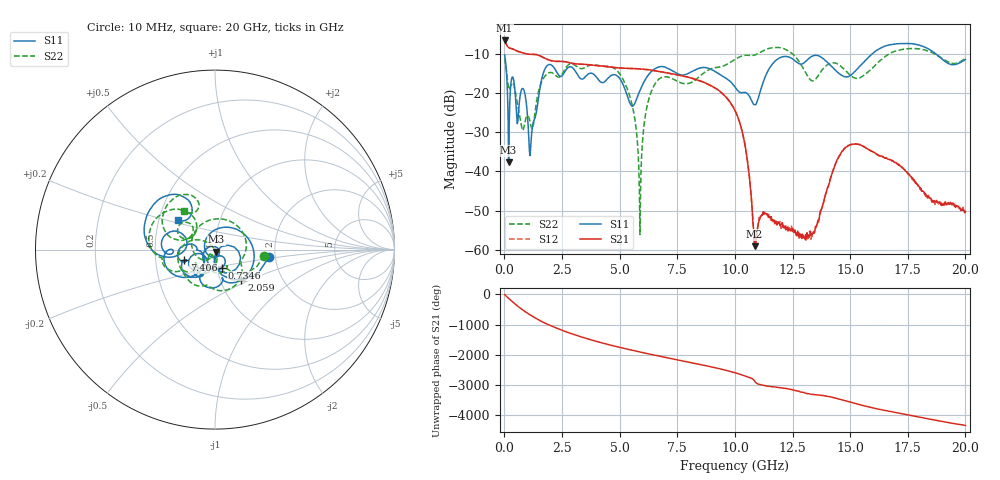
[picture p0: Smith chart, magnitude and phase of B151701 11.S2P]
!  2-Port S-parameters saved by WinCal
! VAR MeasName=S-Parameters (CALIBRATED_DATA) read from VNA (N5244A)
! VAR MeasDate=2015-12-24 19:09:20
! VAR NAME=B151701 11
! VAR FILENAME=B151701 11.S2P
! VAR DATE=2015-12-24 19:09:20
! VAR PHYS_PORTS=1,3
# Hz S DB R 50
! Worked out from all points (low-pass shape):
!   801 points, 10 MHz to 20 GHz, reference 50 ohm
!   highest |S21| = -6.67 dB at 10 MHz (marker M1); lowest = -59.0 dB at 10.85 GHz (marker M2)
!   |S21| within 3 dB of the highest: start of sweep to 710.2 MHz
!   lowest |S11| = -37.7 dB at 184.9 MHz (marker M3), VSWR 1.03, Z = 50.7 - j1.11 ohm
!   |S11| at or under -10 dB: start of sweep to 15.97 GHz; 18.7 GHz to end of sweep
!   |S22| runs from -56.1 to -8.4 dB; largest |S21 - S12| = 0.0011
!   S11 on the Smith chart (normalised r, x): 10 MHz: 1.84, -0.18; 734.6 MHz: 1.06, -0.21; 2.059 GHz: 1.26, -0.45; 7.406 GHz: 0.70, -0.08; 20 GHz: 0.63, +0.22
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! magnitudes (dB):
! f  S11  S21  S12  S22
! 10 MHz  -10.4  -6.7  -6.7  -11.2
! 184.9 MHz  -37.7  -8.4  -8.4  -18.7
! 359.8 MHz  -15.9  -8.8  -8.8  -17.5
! 734.6 MHz  -19.3  -9.7  -9.7  -28.2
! 1.134 GHz  -34.5  -10.2  -10.2  -27.8
! 1.684 GHz  -15.1  -11.0  -11.0  -16.4
! 2.059 GHz  -13.0  -11.8  -11.8  -14.9
! 3.358 GHz  -16.5  -12.7  -12.7  -13.9
! 5.107 GHz  -17.4  -13.7  -13.7  -16.1
! 5.582 GHz  -23.3  -13.8  -13.8  -24.2
! 5.882 GHz  -19.4  -13.9  -13.9  -56.1
! 6.182 GHz  -16.0  -14.1  -14.1  -23.6
! 6.682 GHz  -13.5  -14.5  -14.5  -16.6
! 7.406 GHz  -14.8  -15.3  -15.3  -16.7
! 10.01 GHz  -18.5  -24.5  -24.5  -11.5
! 10.48 GHz  -20.0  -34.7  -34.8  -10.4
! 10.85 GHz  -23.0  -59.0  -58.5  -10.4
! 11.8 GHz  -11.6  -53.2  -53.5  -8.4
! 13.35 GHz  -10.6  -56.0  -56.6  -16.9
! 14.8 GHz  -15.9  -33.9  -33.9  -14.4
! 16.68 GHz  -7.8  -37.0  -36.8  -10.1
! 20 GHz  -11.5  -50.2  -50.5  -11.2
